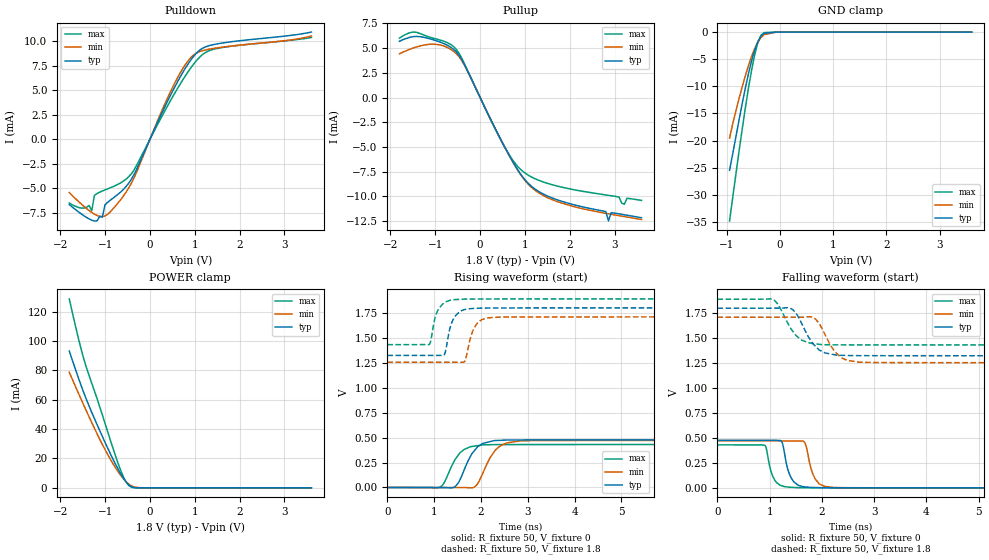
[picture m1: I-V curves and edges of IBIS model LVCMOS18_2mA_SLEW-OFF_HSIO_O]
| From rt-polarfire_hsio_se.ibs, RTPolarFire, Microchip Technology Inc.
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|   Model LVCMOS18_2mA_SLEW-OFF_HSIO_O
[Model]   LVCMOS18_2mA_SLEW-OFF_HSIO_O
Model_type   Output
Polarity   Non-Inverting
Enable   Active-High
Vmeas =   0.9
Cref =   5p
Rref =   1M
|   typ   min   max
C_comp_pullup   1.335e-12   1.335e-12   1.380e-12
C_comp_pulldown  1.335e-12   1.335e-12   1.380e-12
[Temperature Range]  25C   125C   -55C
[Voltage Range]  1.8   1.71   1.89
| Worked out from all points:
|   slope of the pulldown table from 0 to 0.27 V, typ, clamps not added: 99.7 ohm
|   slope of the pullup table from 0 to 0.27 V, typ, clamps not added: 106 ohm
|   GND clamp passes 1 mA (typ) near -0.37 V on its own axis
|   POWER clamp passes 1 mA (typ) near -0.43 V on its own axis
|   rising waveform, R_fixture 50, V_fixture 0: 20-80 % time 313ps typ, 320ps min, 293ps max; typ from 0 V to 0.477 V
|   rising waveform, R_fixture 50, V_fixture 1.8: 20-80 % time 169ps typ, 178ps min, 161ps max; typ from 1.32 V to 1.8 V
|   falling waveform, R_fixture 50, V_fixture 0: 20-80 % time 145ps typ, 149ps min, 134ps max; typ from 0.477 V to 0 V
|   falling waveform, R_fixture 50, V_fixture 1.8: 20-80 % time 319ps typ, 309ps min, 308ps max; typ from 1.8 V to 1.32 V
[GND Clamp]
| Voltage   I(typ)   I(min)   I(max)
-945mV    -25.47mA   -19.54mA   -34.82mA
-885.9mV  -22.44mA   -16.92mA   -30.49mA
-708.7mV  -13.24mA   -10.14mA   -17.96mA
-649.7mV  -10.37mA   -8.095mA   -14.06mA
-590.6mV  -7.705mA   -6.193mA   -10.39mA
-531.6mV  -5.322mA   -4.488mA   -7.054mA
-472.5mV  -3.308mA   -3.028mA   -4.171mA
-413.4mV  -1.757mA   -1.859mA   -1.935mA
-354.4mV  -739.5uA   -1.008mA   -580.7uA
-295.3mV  -232.3uA   -469.6uA   -100.4uA
-59.06mV  -489.8nA   -5.037uA   -176.4nA
3.6V      0A         0A         0A
[POWER Clamp]
| Voltage   I(typ)   I(min)   I(max)
-1.8V     93.11mA    78.61mA    128.6mA
-1.595V   74.64mA    64.3mA     101.4mA
-1.477V   64.73mA    56.23mA    87.68mA
-1.417V   60.07mA    52.24mA    81.73mA
-1.181V   43.06mA    36.84mA    60.8mA
-1.004V   31.04mA    26.13mA    43.96mA
-708.7mV  12.62mA    10.87mA    16.4mA
-590.6mV  6.476mA    6.104mA    7.295mA
-472.5mV  1.932mA    2.452mA    1.539mA
-354.4mV  154uA      598.2uA    74.19uA
-59.06mV  800.7nA    2.877uA    466.9nA
3.6V      0A         0A         0A
[Pullup]
| Voltage   I(typ)   I(min)   I(max)
-1.8V     5.683mA    4.42mA     6.001mA
-1.477V   6.161mA    5.029mA    6.62mA
-1.063V   5.858mA    5.393mA    6.019mA
-531.6mV  4.619mA    4.431mA    4.863mA
562.5mV   -5.136mA   -5.145mA   -5.114mA
1.012V    -8.382mA   -8.455mA   -7.676mA
1.631V    -10.2mA    -10.37mA   -8.849mA
2.804V    -11.53mA   -11.72mA   -9.854mA
2.863V    -12.49mA   -11.77mA   -9.895mA
2.922V    -11.65mA   -11.81mA   -9.936mA
3.217V    -11.86mA   -12.04mA   -10.79mA
3.6V      -12.16mA   -12.34mA   -10.41mA
[Pulldown]
| Voltage   I(typ)   I(min)   I(max)
-1.8V     -6.662mA   -5.438mA   -6.504mA
-1.299V   -8.251mA   -7.462mA   -7.289mA
-1.24V    -8.335mA   -7.633mA   -5.726mA
-1.181V   -8.326mA   -7.771mA   -5.536mA
-1.063V   -7.941mA   -7.889mA   -5.278mA
-885.9mV  -6.219mA   -7.401mA   -4.953mA
-354.4mV  -3.582mA   -3.922mA   -3.118mA
562.5mV   5.408mA    5.812mA    4.769mA
843.8mV   7.63mA     7.949mA    6.831mA
1.125V    9.124mA    8.952mA    8.434mA
1.575V    9.769mA    9.354mA    9.308mA
3.6V      10.92mA    10.51mA    10.36mA
[Ramp]
dV/dt_r   0.286369/0.313004n  0.282788/0.320371n  0.258524/0.292877n
dV/dt_f   0.285972/0.318969n  0.273394/0.308573n  0.275189/0.308364n
R_load = 50
[Rising Waveform]
R_fixture = 50
V_fixture = 0
V_fixture_min = 0
V_fixture_max = 0
| Time   V(typ)   V(min)   V(max)
0s        3.09uV     5.598uV    5.106uV
1.102ns   -618.5uV   -619.4uV   -427.6uV
1.227ns   -689uV     -690.3uV   59.33mV
1.444ns   5.878mV    -813.4uV   278mV
1.64ns    174.5mV    -924.5uV   381mV
1.873ns   376.8mV    8.448mV    415.5mV
2.284ns   469.9mV    359.1mV    429.3mV
2.549ns   475.3mV    446.6mV    430mV
2.843ns   476.2mV    467.6mV    430mV
10ns      477.3mV    471.3mV    430.9mV
[Rising Waveform]
R_fixture = 50
V_fixture = 1.8
V_fixture_min = 1.71
V_fixture_max = 1.89
| Time   V(typ)   V(min)   V(max)
0s        1.323V     1.254V     1.431V
897ps     1.323V     1.254V     1.434V
1.044ns   1.323V     1.255V     1.738V
1.2ns     1.324V     1.255V     1.844V
1.348ns   1.614V     1.255V     1.876V
1.44ns    1.709V     1.255V     1.883V
1.646ns   1.782V     1.26V      1.887V
1.841ns   1.794V     1.585V     1.888V
2.138ns   1.798V     1.698V     1.889V
10ns      1.8V       1.71V      1.89V
[Falling Waveform]
R_fixture = 50
V_fixture = 0
V_fixture_min = 0
V_fixture_max = 0
| Time   V(typ)   V(min)   V(max)
0s        477.3mV    471.3mV    430.9mV
908ps     476.9mV    470.8mV    425.8mV
1.06ns    476.8mV    470.7mV    115.1mV
1.214ns   472.7mV    470.6mV    24.14mV
1.245ns   446.3mV    470.6mV    18.65mV
1.405ns   106.4mV    470.5mV    5.589mV
1.653ns   10.03mV    464.7mV    1.84mV
1.869ns   3.007mV    91.03mV    866.9uV
2.211ns   999.3uV    4.385mV    830.6uV
10ns      4.458uV    7.459uV    4.927uV
[Falling Waveform]
R_fixture = 50
V_fixture = 1.8
V_fixture_min = 1.71
V_fixture_max = 1.89
| Time   V(typ)   V(min)   V(max)
0s        1.8V       1.71V      1.89V
1.058ns   1.801V     1.71V      1.889V
1.153ns   1.801V     1.71V      1.844V
1.398ns   1.799V     1.711V     1.603V
1.61ns    1.651V     1.711V     1.482V
1.816ns   1.452V     1.71V      1.448V
2.003ns   1.367V     1.596V     1.435V
2.243ns   1.334V     1.367V     1.433V
2.695ns   1.325V     1.26V      1.432V
10ns      1.323V     1.254V     1.431V
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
